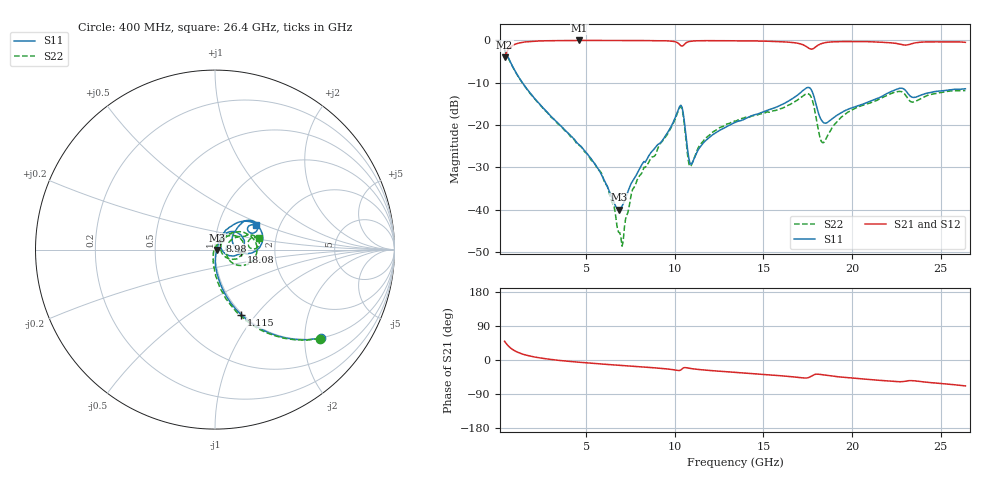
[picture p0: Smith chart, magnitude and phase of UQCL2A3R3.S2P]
! AVX Corporation
! Date:  10/27/06
! Part No:  UQCL2A3R3
! Description:  Ultra Low ESR Microwave capacitors
! Mounting Orientation:  Horizontal
# GHZ S DB R 50
! Freq  |S11|  S11 Ph  |S21|  S21 Ph  |S12|  S12 Ph  |S22|  S22 Ph
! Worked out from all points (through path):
!   401 points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, 400 MHz to 26.4 GHz, reference 50 ohm
!   highest |S21| = -0.03 dB at 4.625 GHz (marker M1); lowest = -4.0 dB at 400 MHz (marker M2)
!   group delay of S21, straight-line fit = 8.42 ps
!   lowest |S11| = -40.0 dB at 6.835 GHz (marker M3), VSWR 1.02, Z = 51 - j0.274 ohm
!   |S11| at or under -10 dB: 1.404 GHz to end of sweep
!   |S22| runs from -48.6 to -2.3 dB; largest |S21 - S12| = 0.0018
!   S11 on the Smith chart (normalised r, x): 400 MHz: 1.00, -2.40; 1.115 GHz: 0.98, -0.85; 8.98 GHz: 1.05, +0.11; 18.08 GHz: 1.34, -0.04; 26.4 GHz: 1.52, +0.45
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0.4  -2.28 -39.8  -3.96 49.4  -3.96 49.4  -2.31 -40.4
1.115  -8.13 -68.0  -0.75 20.9  -0.75 20.9  -8.19 -69.4
4.625  -24.73 -87.5  -0.03 -6.0  -0.03 -6.0  -24.81 -100.5
4.755  -25.25 -87.8  -0.04 -6.6  -0.04 -6.6  -25.31 -100.5
6.12  -33.85 -71.7  -0.04 -11.5  -0.04 -11.5  -34.01 -118.4
6.835  -39.98 -15.5  -0.04 -13.9  -0.04 -13.9  -45.33 -168.4
7.03  -39.10 11.0  -0.04 -14.5  -0.04 -14.5  -48.59 151.3
7.68  -32.85 46.7  -0.04 -16.7  -0.03 -16.7  -34.83 78.7
8.98  -24.89 61.8  -0.10 -21.0  -0.10 -21.0  -26.31 60.2
9.11  -24.41 60.6  -0.09 -21.4  -0.09 -21.4  -24.85 60.3
10.28  -15.57 29.2  -1.00 -27.6  -1.00 -27.5  -15.86 17.4
10.93  -29.28 20.6  -0.20 -22.6  -0.21 -22.6  -29.52 16.6
11.775  -23.56 59.2  -0.08 -26.9  -0.08 -26.9  -22.96 49.5
13.4  -19.38 62.2  -0.12 -32.6  -0.11 -32.6  -19.06 48.9
16.91  -12.99 44.8  -0.66 -45.7  -0.66 -45.7  -14.14 27.1
17.755  -12.08 2.8  -2.07 -41.4  -2.06 -41.4  -14.00 -24.4
18.08  -16.78 -5.6  -1.16 -37.4  -1.16 -37.4  -20.67 -35.2
18.405  -19.45 14.0  -0.63 -39.4  -0.63 -39.4  -24.12 3.5
19.705  -16.42 42.5  -0.29 -46.4  -0.29 -46.4  -17.14 29.7
22.11  -12.28 42.0  -0.56 -55.6  -0.56 -55.6  -12.73 19.6
23.475  -13.48 29.4  -0.68 -54.7  -0.68 -54.8  -14.55 10.5
26.4  -11.44 30.8  -0.47 -68.5  -0.47 -68.4  -11.86 14.2
